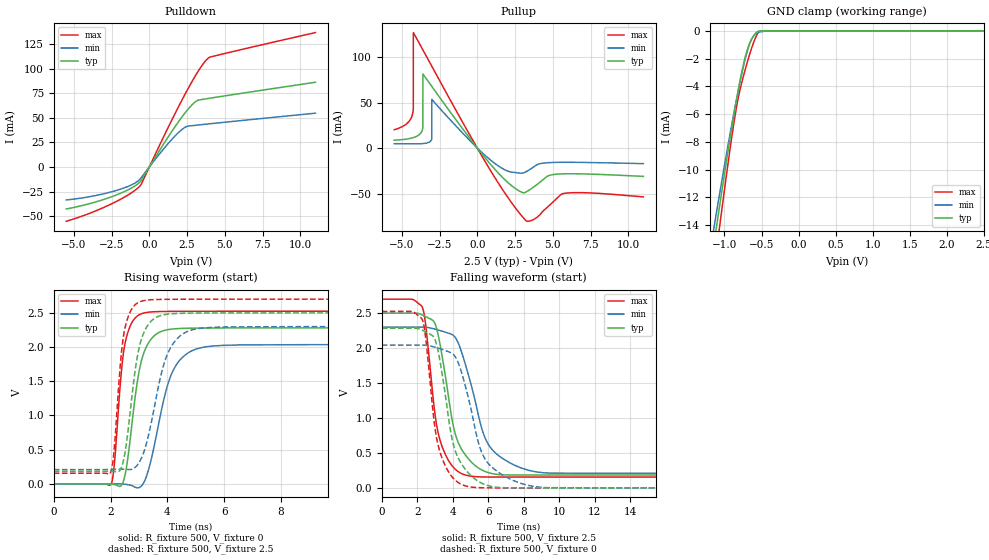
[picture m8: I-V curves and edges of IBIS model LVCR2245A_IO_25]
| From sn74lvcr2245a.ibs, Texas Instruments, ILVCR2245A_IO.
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[Model]   LVCR2245A_IO_25
Model_type  I/O
Vinl=0.7
Vinh=1.7
Enable   Active-Low
Vref =   0
Rref =   500
Cref =   30p
Vmeas =   1.25
| variable   typ   min   max
C_comp   5.76pF   5.50pF   6.25pF
| C_pullup   4.99pF   4.43pF   6.30pF
| C_pulldown   4.38pF   3.92pF   5.46pF
| C_tri-state   5.76pF   5.50pF   6.25pF
[Temperature Range]   40   100   -40
| Ambient temperature   25   85   -40
[Voltage range]   2.5   2.3   2.7
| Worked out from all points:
|   slope of the pulldown table from 0 to 0.375 V, typ, clamps not added: 39.8 ohm
|   slope of the pullup table from 0 to 0.375 V, typ, clamps not added: 47.9 ohm
|   GND clamp passes 1 mA (typ) near -0.67 V on its own axis
|   rising waveform, R_fixture 500, V_fixture 0: 20-80 % time 470ps typ, 712ps min, 317ps max; typ from 0 V to 2.28 V
|   falling waveform, R_fixture 500, V_fixture 2.5: 20-80 % time 1.02ns typ, 1.42ns min, 768ps max; typ from 2.5 V to 0.183 V
|   rising waveform, R_fixture 500, V_fixture 2.5: 20-80 % time 457ps typ, 703ps min, 309ps max; typ from 0.183 V to 2.5 V
|   falling waveform, R_fixture 500, V_fixture 0: 20-80 % time 981ps typ, 1.32ns min, 763ps max; typ from 2.28 V to 0 V
[GND Clamp]
| LVCR2245A_IO_25
|   Voltage   I(typ)   I(min)   I(max)
-5.5V     -191mA     -172.6mA   -219.2mA
-1.155V   -15.81mA   -14.6mA    -17.82mA
-1.115V   -14.36mA   -13.31mA   -16.15mA
-1.08V    -13.11mA   -12.19mA   -14.7mA
-1.045V   -11.88mA   -11.09mA   -13.26mA
-930mV    -7.937mA   -7.574mA   -8.711mA
-850mV    -5.367mA   -5.277mA   -5.881mA
-745mV    -2.448mA   -2.581mA   -3.287mA
-690mV    -1.345mA   -1.427mA   -2.227mA
-635mV    -627.2uA   -606.9uA   -1.272mA
-525mV    -20.03uA   -86.68uA   -33.12uA
2.5V      50.36pA    25.99nA    -1.56nA
[Pulldown]
| LVCR2245A_IO_25
|   Voltage   I(typ)   I(min)   I(max)
-5.5V     -42.76mA   -33.57mA   -55.31mA
-3.855V   -36.9mA    -29.98mA   -46.61mA
-2.35V    -29.48mA   -24.64mA   -36.38mA
-1.21V    -21.69mA   -18.45mA   -26.57mA
-620mV    -15.21mA   -12.36mA   -19.37mA
1.09V     26.86mA    21.04mA    35.29mA
2.155V    50.78mA    38.04mA    67.95mA
2.515V    57.89mA    41.42mA    78.36mA
3.09V     66.82mA    42.47mA    93.87mA
3.57V     68.9mA     43.26mA    105.1mA
3.92V     69.76mA    43.82mA    111mA
11V       86.22mA    54.74mA    136.8mA
[Pullup]
| LVCR2245A_IO_25
|   Voltage   I(typ)   I(min)   I(max)
-5.5V     8.675mA    4.847mA    20.15mA
-4.27V    11.34mA    4.729mA    38.41mA
-4.235V   11.52mA    4.726mA    43.18mA
-4.23V    11.54mA    4.725mA    126.9mA
-3.615V   21.4mA     4.95mA     108.3mA
-3.605V   22.84mA    4.964mA    108mA
-3.6V     81.41mA    4.971mA    107.8mA
-3.02V    67.99mA    9.734mA    90.18mA
-3.01V    67.76mA    53.49mA    89.87mA
3.235V    -48.18mA   -25.9mA    -79.88mA
5.73V     -28.24mA   -15.62mA   -49.77mA
11V       -31.06mA   -17.08mA   -53.61mA
[Ramp]
| LVCR2245A_IO_25
| variable   typ   min   max
dV/dt_r   1.39/4.81E-10   1.26/7.29E-10   1.53/3.23E-10
dV/dt_f   1.39/1.02E-09   1.26/1.43E-09   1.53/7.71E-10
R_load = 500
[Rising Waveform]
| LVCR2245A_IO_25
R_fixture =   500
C_fixture =   0
L_fixture =   0
V_fixture =   0
V_fixture_min = 0
V_fixture_max = 0
|   Time   V(typ)   V(min)   V(max)
0s        793.1pV    2.962nV    26.69nV
2.03ns    -2.917mV   -691.3uV   6.217mV
2.145ns   -12.09mV   -515.2uV   341.6mV
2.39ns    -18.55mV   -1.365mV   1.679V
2.52ns    149.8mV    -6.542mV   2.073V
2.985ns   1.598V     -57.11mV   2.465V
3.335ns   2.059V     202mV      2.509V
4.215ns   2.264V     1.666V     2.521V
5.565ns   2.278V     2.014V     2.522V
50ns      2.281V     2.036V     2.523V
[Falling Waveform]
| LVCR2245A_IO_25
R_fixture =   500
C_fixture =   0
L_fixture =   0
V_fixture =   2.5
V_fixture_min = 2.3
V_fixture_max = 2.7
|   Time   V(typ)   V(min)   V(max)
0s        2.5V       2.3V       2.7V
2.29ns    2.474V     2.301V     2.584V
2.49ns    2.448V     2.299V     2.298V
2.945ns   2.376V     2.275V     1.168V
3.33ns    1.989V     2.247V     642.8mV
4.095ns   817.9mV    2.167V     278mV
4.885ns   414.3mV    1.614V     173mV
6.11ns    210.4mV    583.3mV    155.2mV
8.9ns     183.6mV    221.7mV    154.8mV
50ns      183.5mV    208.7mV    154.7mV
[Rising Waveform]
| LVCR2245A_IO_25
R_fixture =   500
C_fixture =   0
L_fixture =   0
V_fixture =   2.5
V_fixture_min = 2.3
V_fixture_max = 2.7
|   Time   V(typ)   V(min)   V(max)
0s        183.5mV    208.6mV    154.6mV
1.995ns   186.1mV    209.8mV    160.6mV
2.11ns    182.6mV    211.5mV    431.7mV
2.35ns    209.2mV    215.1mV    1.77V
2.495ns   424.5mV    213.4mV    2.253V
2.945ns   1.864V     274.9mV    2.643V
3.285ns   2.301V     623.5mV    2.686V
4.075ns   2.483V     1.959V     2.697V
5.315ns   2.497V     2.281V     2.699V
50ns      2.5V       2.3V       2.7V
[Falling Waveform]
| LVCR2245A_IO_25
R_fixture =   500
C_fixture =   0
L_fixture =   0
V_fixture =   0
V_fixture_min = 0
V_fixture_max = 0
|   Time   V(typ)   V(min)   V(max)
0s        2.283V     2.042V     2.524V
2.29ns    2.256V     2.043V     2.405V
2.935ns   2.155V     2.017V     984.8mV
3.31ns    1.772V     1.989V     489.9mV
4.03ns    626.3mV    1.91V      137.9mV
4.88ns    213.1mV    1.288V     18.24mV
5.475ns   88.26mV    621.3mV    2.939mV
5.96ns    34.2mV     362.1mV    731.8uV
8.82ns    134uV      11.61mV    170.4uV
50ns      24.99uV    69.87uV    8.467uV
